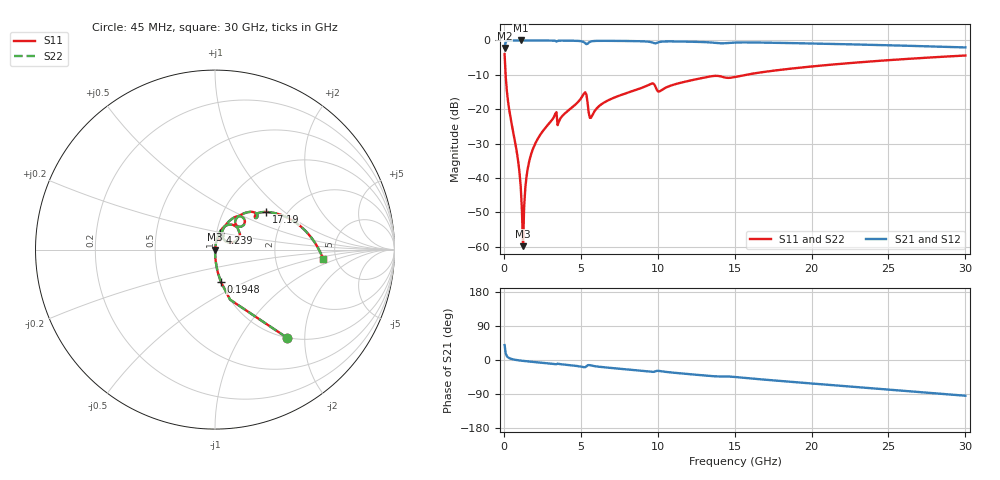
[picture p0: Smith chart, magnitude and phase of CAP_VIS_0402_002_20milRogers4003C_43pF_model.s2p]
! S-parameter model data by Modelithics Inc.  support@modelithics.com  813-866-6335  Tampa FL USA
! S-Parameter data specifications:
! Substrate: 20-mil Rogers 4003C, substrate thickness, H=0.508mm, Dielectric constant, Er=3.75
! PCB Mounting Pad Footprint: Pad width, PadW=0.50mm , Pad length, PadL=0.50mm , Pad gap, PadG (edge-to-edge)=0.40mm , Reference planes=1.4mm apart
! Created Wed Nov 18 12:55:15 2015
# hz S ma R 50
! 2 Port Network Data from SP1.SP block
! freq  magS11  angS11  magS21  angS21  magS12  angS12  magS22  angS22
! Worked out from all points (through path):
!   401 points, 45 MHz to 30 GHz, reference 50 ohm
!   highest |S21| = -0.01 dB at 1.093 GHz (marker M1); lowest = -2.2 dB at 45 MHz (marker M2)
!   group delay of S21, straight-line fit = 8.89 ps
!   lowest |S11| = -59.8 dB at 1.243 GHz (marker M3), VSWR 1.00, Z = 50.1 + j0.0292 ohm
!   |S11| at or under -10 dB: 112 MHz to 15.73 GHz (15.61 GHz wide, 197 % of centre)
!   |S22| runs from -59.8 to -4.0 dB; largest |S21 - S12| = 0
!   S11 on the Smith chart (normalised r, x): 45 MHz: 1.00, -1.63; 194.8 MHz: 1.00, -0.37; 4.239 GHz: 1.03, +0.20; 17.19 GHz: 1.58, +0.76; 30 GHz: 3.94, -0.62
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4.5e7  0.6333 -50.8  0.7737 39.2  0.7737 39.2  0.6333 -50.8
1.94775e8  0.1815 -79.8  0.983 10.1  0.983 10.1  0.1815 -79.8
3.4455e8  0.09824 -84.7  0.9946 5.0  0.9946 5.0  0.09824 -84.7
8.687625e8  0.02155 -88.2  0.9989 -0.4  0.9989 -0.4  0.02155 -88.2
1.093425e9  0.007432 -84.6  0.999 -1.6  0.999 -1.6  0.007432 -84.6
1.2432e9  0.001021 16.6  0.999 -2.3  0.999 -2.3  0.001021 16.6
1.392975e9  0.007255 78.9  0.9989 -3.0  0.9989 -3.0  0.007255 78.9
1.617638e9  0.01643 82.2  0.9987 -3.9  0.9987 -3.9  0.01643 82.2
2.066962e9  0.03265 82.1  0.9981 -5.7  0.9981 -5.7  0.03265 82.1
3.265162e9  0.07827 76.3  0.9925 -10.5  0.9925 -10.5  0.07827 76.3
3.6396e9  0.07128 75.9  0.9933 -10.8  0.9933 -10.8  0.07128 75.9
4.2387e9  0.09794 74.8  0.9921 -13.5  0.9921 -13.5  0.09794 74.8
5.062462e9  0.1497 64.6  0.9691 -17.9  0.9691 -17.9  0.1497 64.6
5.287125e9  0.176 45.1  0.9099 -18.9  0.9099 -18.9  0.176 45.1
5.661562e9  0.07525 51.3  0.9665 -14.4  0.9665 -14.4  0.07525 51.3
9.480825e9  0.2297 54.3  0.9535 -30.8  0.9535 -30.8  0.2297 54.3
1.007992e10  0.1804 48.7  0.9451 -28.8  0.9451 -28.8  0.1804 48.7
1.50225e10  0.2939 40.5  0.9319 -44.9  0.9319 -44.9  0.2939 40.5
1.719424e10  0.3553 36.1  0.9272 -52.7  0.9272 -52.7  0.3553 36.1
2.003996e10  0.4188 27.2  0.9022 -62.1  0.9022 -62.1  0.4188 27.2
2.505742e10  0.5175 11.2  0.8498 -78.3  0.8498 -78.3  0.5175 11.2
3e10  0.6037 -4.8  0.7909 -94.3  0.7909 -94.3  0.6037 -4.8
